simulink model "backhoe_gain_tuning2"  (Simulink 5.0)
settings: Solver=ode4  StartTime=0.0  StopTime=inf  FixedStep=0.001  RelTol=1e-3
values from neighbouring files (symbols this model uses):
  Butter_Order = 2    [startup.m]
  c1 = [-0.0009634 -0.4050766 2.3355377]    [startup.m]
  c2 = [ -0.00644514 2.23812750 22.79925627]    [startup.m]
  c3 = [-0.0057802 2.2376391 22.8266324]    [startup.m]
  c4 = [-0.0020828 1.5286223 20.3434998]    [startup.m]
undefined symbols (not defined in the file or in its folder): channels, ended, Single
libraries: dsparch4 x18, xpclib x6, simulink x1

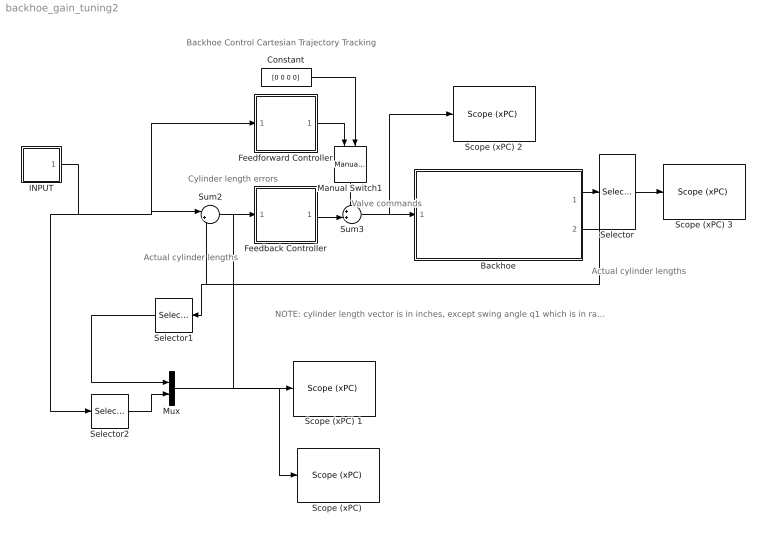
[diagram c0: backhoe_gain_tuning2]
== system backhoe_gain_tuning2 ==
  note: Backhoe Control Cartesian Trajectory Tracking
  note: NOTE: cylinder length vector is in inches, except swing angle q1 which is in radians: yc = [ q1[rad] yc,boom[in] yc,stick[in] yc,bucket[in] ]^T
  note: Cylinder length errors
  note: Actual cylinder lengths
  note: Actual cylinder lengths
  note: Valve commands
  Backhoe : Subsystem
  Constant : Constant  Value=[0 0 0 0]
  Feedback Controller : Subsystem
  Feedforward Controller : Subsystem
  INPUT : Subsystem
  Manual Switch1 : simulink/Signal Routing/Manual Switch  Orientation=down  sw=1  action=0
  Mux : Mux  Inputs=2
  "Scope (xPC) " : xpclib/Misc./Scope (xPC)   scopeno=1  scopetype=Target  viewmode=Graphical redraw  grid=on  ylimits=[0,40]  autostart=on  nosamples=2000  noprepostsamples=0  interleave=1  triggermode=FreeRun  triggersignal=1  triggerlevel=0.0  triggerslope=either  triggerscope=1  triggersample=0
  Scope (xPC) 1 : xpclib/Misc./Scope (xPC)   scopeno=2  scopetype=Target  viewmode=Graphical redraw  grid=on  ylimits=[-3,3]  autostart=on  nosamples=2000  noprepostsamples=0  interleave=1  triggermode=FreeRun  triggersignal=1  triggerlevel=0.0  triggerslope=either  triggerscope=1  triggersample=0
  Scope (xPC) 2 : xpclib/Misc./Scope (xPC)   scopeno=3  scopetype=Target  viewmode=Graphical redraw  grid=on  ylimits=[-1,1]  autostart=on  nosamples=2000  noprepostsamples=0  interleave=1  triggermode=FreeRun  triggersignal=1  triggerlevel=0.0  triggerslope=either  triggerscope=1  triggersample=0
  Scope (xPC) 3 : xpclib/Misc./Scope (xPC)   scopeno=4  scopetype=Target  viewmode=Graphical redraw  grid=on  ylimits=[0,1000]  autostart=on  nosamples=2000  noprepostsamples=0  interleave=1  triggermode=FreeRun  triggersignal=1  triggerlevel=0.0  triggerslope=either  triggerscope=1  triggersample=0
  Selector : Selector  Elements=[3 7]  InputPortWidth=10
  Selector1 : Selector  Orientation=left  Elements=[3]  InputPortWidth=4
  Selector2 : Selector  Elements=[3]  InputPortWidth=4
  Sum2 : Sum  Inputs=|+-
  Sum3 : Sum  Inputs=++|
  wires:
  Sum2/1 -> Feedback Controller/1(e), Scope (xPC) 1/1
  Backhoe/2(yc) -> Sum2/2, Selector1/1
  Feedback Controller/1(Us) -> Sum3/2
  Sum3/1 -> Backhoe/1(Us), Scope (xPC) 2/1
  Manual Switch1/1 -> Sum3/1
  Feedforward Controller/1(UsFF) -> Manual Switch1/1
  Constant/1 -> Manual Switch1/2
  Mux/1 -> "Scope (xPC) "/1
  Selector2/1 -> Mux/2
  Selector1/1 -> Mux/1
  INPUT/1(ycdes) -> Selector2/1, Sum2/1, Feedforward Controller/1(ycdes)
  Backhoe/1(Pres) -> Selector/1
  Selector/1 -> Scope (xPC) 3/1

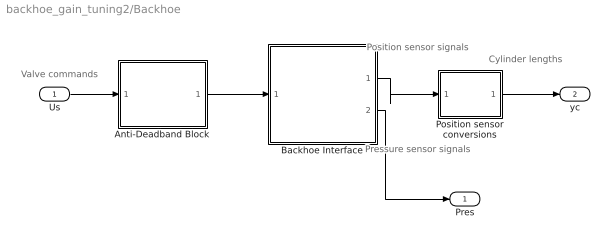
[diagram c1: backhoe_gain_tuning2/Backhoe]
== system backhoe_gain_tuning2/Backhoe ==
  note: Valve commands
  note: Position sensor signals
  note: Cylinder lengths
  note: Pressure sensor signals
  Us : Inport
  Anti-Deadband Block : Subsystem
  Backhoe Interface : Subsystem
  Position sensor conversions : Subsystem
  Pres : Outport
  yc : Outport  Port=2
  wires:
  Backhoe Interface/1(Vpos) -> Position sensor conversions/1(Vc)
  Position sensor conversions/1(yc) -> yc/1
  Us/1 -> Anti-Deadband Block/1(us)
  Backhoe Interface/2(Vpres) -> Pres/1
  Anti-Deadband Block/1(Us) -> Backhoe Interface/1(Us)

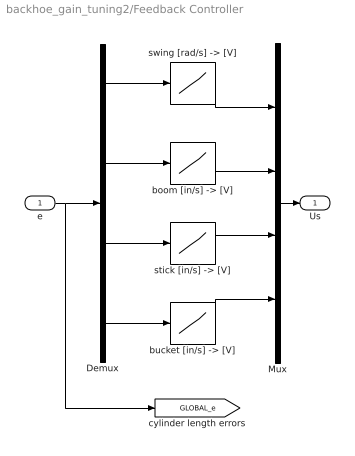
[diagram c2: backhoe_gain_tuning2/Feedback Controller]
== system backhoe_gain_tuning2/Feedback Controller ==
  e : Inport
  Demux : Demux
  Mux : Mux
  "boom [in/s] -> [V]" : Lookup  InputValues=[-1 0 1]  OutputValues=[-0.05 0 0.6]  ShowAdditionalParam=on
  "bucket [in/s] -> [V]" : Lookup  InputValues=[-1 0 1]  OutputValues=[-0.2 0 0.2]  ShowAdditionalParam=on
  "stick [in/s] -> [V]" : Lookup  InputValues=[-1 0 1]  OutputValues=[-0.2 0 0.2]  ShowAdditionalParam=on
  "swing [rad/s] -> [V]" : Lookup  InputValues=[-1 0 1]  OutputValues=[-0.2 0 0.2]  ShowAdditionalParam=on
  Us : Outport
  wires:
  e/1 -> [GLOBAL_e], Demux/1
  Demux/1 -> "swing [rad/s] -> [V]"/1
  "swing [rad/s] -> [V]"/1 -> Mux/1
  Demux/2 -> "boom [in/s] -> [V]"/1
  "boom [in/s] -> [V]"/1 -> Mux/2
  Demux/3 -> "stick [in/s] -> [V]"/1
  "stick [in/s] -> [V]"/1 -> Mux/3
  Demux/4 -> "bucket [in/s] -> [V]"/1
  "bucket [in/s] -> [V]"/1 -> Mux/4
  Mux/1 -> Us/1

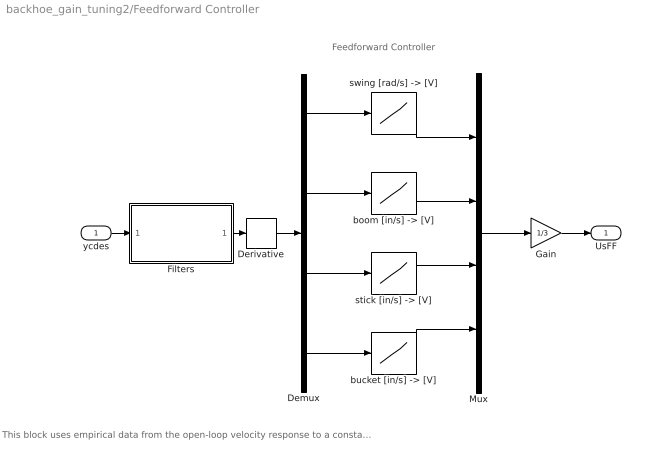
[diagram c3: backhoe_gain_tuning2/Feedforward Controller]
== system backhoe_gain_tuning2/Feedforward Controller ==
  note: This block uses empirical data from the open-loop velocity response to a constant voltage command to the valves. Relationships have been inverted to determine the required voltage to produce a desired velocity for each function.
  note: Feedforward Controller
  ycdes : Inport
  Demux : Demux
  Derivative : Derivative
  Filters : Subsystem
  Gain : Gain  Gain=1/3
  Mux : Mux
  "boom [in/s] -> [V]" : Lookup  InputValues=[-1.0 0 3.0]  OutputValues=[-0.25 0 0.25]  ShowAdditionalParam=on
  "bucket [in/s] -> [V]" : Lookup  InputValues=[-2.3 0 2.75]  OutputValues=[-0.25 0 0.25]  ShowAdditionalParam=on
  "stick [in/s] -> [V]" : Lookup  InputValues=[-1.6 0 1.75]  OutputValues=[-0.25 0 0.25]  ShowAdditionalParam=on
  "swing [rad/s] -> [V]" : Lookup  InputValues=[-0.6 0 0.7]  OutputValues=[-0.25 0 0.25]  ShowAdditionalParam=on
  UsFF : Outport
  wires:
  ycdes/1 -> Filters/1(unfiltered)
  Derivative/1 -> Demux/1
  Demux/1 -> "swing [rad/s] -> [V]"/1
  "swing [rad/s] -> [V]"/1 -> Mux/1
  Demux/2 -> "boom [in/s] -> [V]"/1
  "boom [in/s] -> [V]"/1 -> Mux/2
  Demux/3 -> "stick [in/s] -> [V]"/1
  "stick [in/s] -> [V]"/1 -> Mux/3
  Demux/4 -> "bucket [in/s] -> [V]"/1
  "bucket [in/s] -> [V]"/1 -> Mux/4
  Mux/1 -> Gain/1
  Filters/1(filtered) -> Derivative/1
  Gain/1 -> UsFF/1

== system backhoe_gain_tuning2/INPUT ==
  Boom : Sin  Amplitude=0  Bias=31  Frequency=2*pi*0.1  SampleTime=0
  Bucket : Sin  Amplitude=0  Bias=32  Frequency=2*pi*0.1  SampleTime=0
  Mux2 : Mux
  Stick : Sin  Amplitude=0  Bias=33  Frequency=2*pi*0.1  SampleTime=0
  Swing : Sin  Amplitude=0  Frequency=2*pi*0.1  SampleTime=0
  ycdes : Outport
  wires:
  Swing/1 -> Mux2/1
  Bucket/1 -> Mux2/4
  Stick/1 -> Mux2/3
  Boom/1 -> Mux2/2
  Mux2/1 -> ycdes/1

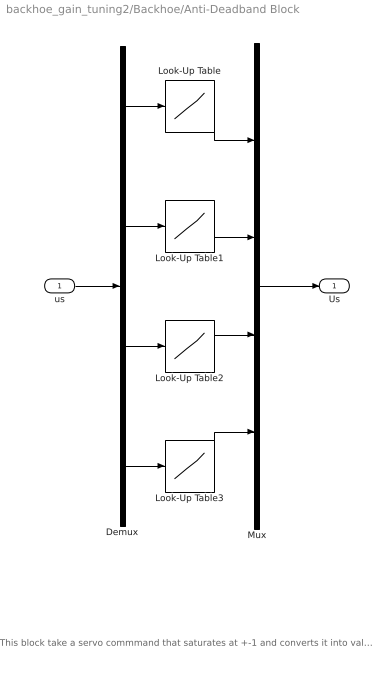
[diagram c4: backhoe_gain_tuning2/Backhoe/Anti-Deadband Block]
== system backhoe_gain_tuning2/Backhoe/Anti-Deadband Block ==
  note: This block take a servo commmand that saturates at +-1 and converts it into valve signals. "u" in the input signal which a 4-vector. Neutral is half the voltage supplied Vc to the valves which should 6V = 1/2 * 12V. Commands to the valve must be between 25% AND 75% of Vc where 50% is neutral or the "zero command" that tell the valve to stop flow to the valve. Neutral can either be set at 6V of measure from Channel 15.
  us : Inport
  Demux : Demux
  Look-Up Table{,1..3} (4 alike) : Lookup  InputValues=[-1 -0.02 0.02 1]  OutputValues=[3 5.45 6.55 9]  ShowAdditionalParam=on  LookUpMeth=Interpolation-Use End Values  OutDataTypeMode=double
  Mux : Mux
  Us : Outport
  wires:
  Look-Up Table/1 -> Mux/1
  Look-Up Table1/1 -> Mux/2
  Demux/1 -> Look-Up Table/1
  Demux/2 -> Look-Up Table1/1
  Demux/3 -> Look-Up Table2/1
  Look-Up Table2/1 -> Mux/3
  Demux/4 -> Look-Up Table3/1
  Look-Up Table3/1 -> Mux/4
  Mux/1 -> Us/1
  us/1 -> Demux/1

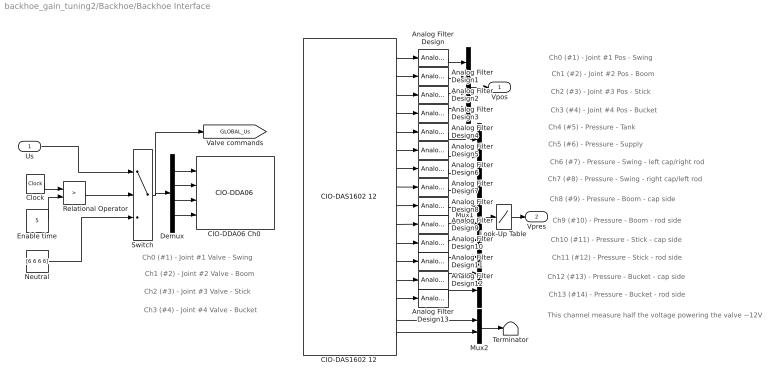
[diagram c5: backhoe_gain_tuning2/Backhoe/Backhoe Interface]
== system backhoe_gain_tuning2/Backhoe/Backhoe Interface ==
  note: Ch0 (#1) - Joint #1 Valve - Swing
  note: Ch1 (#2) - Joint #2 Valve - Boom
  note: Ch2 (#3) - Joint #3 Valve - Stick
  note: Ch3 (#4) - Joint #4 Valve - Bucket
  note: Ch0 (#1) - Joint #1 Pos - Swing
  note: Ch1 (#2) - Joint #2 Pos - Boom
  note: Ch2 (#3) - Joint #3 Pos - Stick
  note: Ch3 (#4) - Joint #4 Pos - Bucket
  note: Ch4 (#5) - Pressure - Tank
  note: Ch5 (#6) - Pressure - Supply
  note: Ch6 (#7) - Pressure - Swing - left cap/right rod
  note: Ch7 (#8) - Pressure - Swing - right cap/left rod
  note: Ch8 (#9) - Pressure - Boom - cap side
  note: Ch9 (#10) - Pressure - Boom - rod side
  note: Ch10 (#11) - Pressure - Stick - cap side
  note: Ch11 (#12) - Pressure - Stick - rod side
  note: Ch12 (#13) - Pressure - Bucket - cap side
  note: Ch13 (#14) - Pressure - Bucket - rod side
  note: This channel measure half the voltage powering the valve ~12V
  Us : Inport
  Analog Filter Design{,1..13} (14 alike) : dsparch4/Analog Filter Design  method=Butterworth  filttype=Lowpass  N=Butter_Order  Wlo=Butter_Rad  Whi=80  Rp=2  Rs=40
  "CIO-DAS1602 12 " : xpclib/A//D/Computer Boards/CIO-DAS1602 12   channel=16  range=0-10V  mux=Single-ended (16 channels)  sampletime=0.001  baseaddress=0x340
  "CIO-DDA06 Ch0 " : xpclib/D//A/Computer Boards/CIO-DDA06   channel=[1 2 3 4]  range=[10 10 10 10]  reset=[1 1 1 1]  initValue=[6 6 6 6]  sampletime=0.001  baseaddress=0x300
  Clock : Clock
  Demux : Demux
  Enable time : Constant  Value=5
  Look-Up Table : Lookup  InputValues=[2 10]  OutputValues=[0 3000]
  Mux : Mux
  Mux1 : Mux  Inputs=10
  Mux2 : Mux  Inputs=2
  Neutral : Constant  Value=[6 6 6 6]  ShowAdditionalParam=on
  Relational Operator : RelationalOperator  Operator=>  ShowAdditionalParam=on
  Switch : Switch  Threshold=0.5  ShowAdditionalParam=on
  Terminator : Terminator
  Vpos : Outport
  Vpres : Outport  Port=2
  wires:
  Demux/1 -> "CIO-DDA06 Ch0 "/1
  Demux/2 -> "CIO-DDA06 Ch0 "/2
  Demux/3 -> "CIO-DDA06 Ch0 "/3
  Demux/4 -> "CIO-DDA06 Ch0 "/4
  Mux/1 -> Vpos/1
  "CIO-DAS1602 12 "/1 -> Analog Filter Design/1
  Analog Filter Design/1 -> Mux/1
  "CIO-DAS1602 12 "/2 -> Analog Filter Design1/1
  "CIO-DAS1602 12 "/3 -> Analog Filter Design2/1
  "CIO-DAS1602 12 "/4 -> Analog Filter Design3/1
  Analog Filter Design1/1 -> Mux/2
  Analog Filter Design2/1 -> Mux/3
  Analog Filter Design3/1 -> Mux/4
  "CIO-DAS1602 12 "/5 -> Analog Filter Design4/1
  "CIO-DAS1602 12 "/6 -> Analog Filter Design5/1
  "CIO-DAS1602 12 "/7 -> Analog Filter Design6/1
  "CIO-DAS1602 12 "/8 -> Analog Filter Design7/1
  "CIO-DAS1602 12 "/9 -> Analog Filter Design8/1
  "CIO-DAS1602 12 "/10 -> Analog Filter Design9/1
  "CIO-DAS1602 12 "/11 -> Analog Filter Design10/1
  "CIO-DAS1602 12 "/12 -> Analog Filter Design11/1
  "CIO-DAS1602 12 "/13 -> Analog Filter Design12/1
  "CIO-DAS1602 12 "/14 -> Analog Filter Design13/1
  "CIO-DAS1602 12 "/15 -> Mux2/1
  Analog Filter Design4/1 -> Mux1/1
  Analog Filter Design5/1 -> Mux1/2
  Analog Filter Design6/1 -> Mux1/3
  Analog Filter Design7/1 -> Mux1/4
  Analog Filter Design8/1 -> Mux1/5
  Analog Filter Design9/1 -> Mux1/6
  Analog Filter Design10/1 -> Mux1/7
  Analog Filter Design11/1 -> Mux1/8
  Analog Filter Design12/1 -> Mux1/9
  Analog Filter Design13/1 -> Mux1/10
  Mux2/1 -> Terminator/1
  "CIO-DAS1602 12 "/16 -> Mux2/2
  Switch/1 -> Demux/1, [GLOBAL_Us]
  Clock/1 -> Relational Operator/1
  Enable time/1 -> Relational Operator/2
  Relational Operator/1 -> Switch/2
  Neutral/1 -> Switch/3
  Us/1 -> Switch/1
  Look-Up Table/1 -> Vpres/1
  Mux1/1 -> Look-Up Table/1

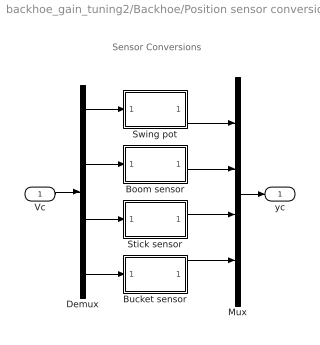
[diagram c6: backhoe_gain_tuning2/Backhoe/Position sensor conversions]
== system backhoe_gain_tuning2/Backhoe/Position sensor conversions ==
  note: Sensor Conversions
  Vc : Inport
  Boom sensor : Subsystem
  Bucket sensor : Subsystem
  Demux : Demux
  Mux : Mux
  Stick sensor : Subsystem
  Swing pot : Subsystem
  yc : Outport
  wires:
  Vc/1 -> Demux/1
  Demux/1 -> Swing pot/1(Vc1)
  Demux/2 -> Boom sensor/1(Vc2)
  Swing pot/1(q1) -> Mux/1
  Boom sensor/1(yc3) -> Mux/2
  Demux/3 -> Stick sensor/1(Vc3)
  Stick sensor/1(yc4) -> Mux/3
  Mux/1 -> yc/1
  Demux/4 -> Bucket sensor/1(Vc4)
  Bucket sensor/1(yc5) -> Mux/4

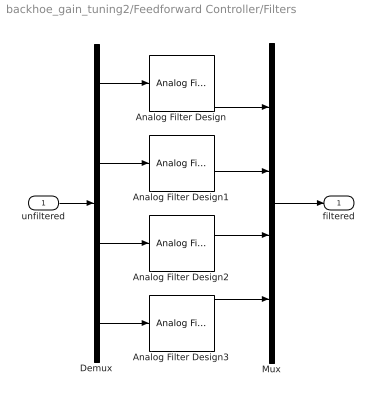
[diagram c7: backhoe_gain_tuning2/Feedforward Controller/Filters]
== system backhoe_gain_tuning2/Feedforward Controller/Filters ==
  unfiltered : Inport
  Analog Filter Design{,1..3} (4 alike) : dsparch4/Analog Filter Design  method=Butterworth  filttype=Lowpass  N=2  Wlo=2*pi*5  Whi=80  Rp=2  Rs=40
  Demux : Demux
  Mux : Mux
  filtered : Outport
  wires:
  unfiltered/1 -> Demux/1
  Demux/1 -> Analog Filter Design/1
  Analog Filter Design/1 -> Mux/1
  Demux/2 -> Analog Filter Design1/1
  Analog Filter Design1/1 -> Mux/2
  Demux/3 -> Analog Filter Design2/1
  Analog Filter Design2/1 -> Mux/3
  Demux/4 -> Analog Filter Design3/1
  Analog Filter Design3/1 -> Mux/4
  Mux/1 -> filtered/1

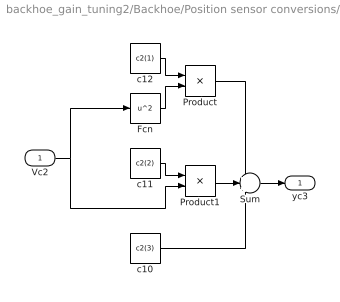
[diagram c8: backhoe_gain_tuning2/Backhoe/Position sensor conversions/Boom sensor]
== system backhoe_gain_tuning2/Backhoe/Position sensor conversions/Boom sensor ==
  Vc2 : Inport
  Fcn : Fcn  Expr=u^2
  Product : Product
  Product1 : Product
  Sum : Sum  Inputs=+++
  c10 : Constant  Value=c2(3)
  c11 : Constant  Value=c2(2)
  c12 : Constant  Value=c2(1)
  yc3 : Outport
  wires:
  Vc2/1 -> Fcn/1, Product1/2
  Product1/1 -> Sum/2
  c10/1 -> Sum/3
  c12/1 -> Product/1
  Fcn/1 -> Product/2
  Product/1 -> Sum/1
  c11/1 -> Product1/1
  Sum/1 -> yc3/1

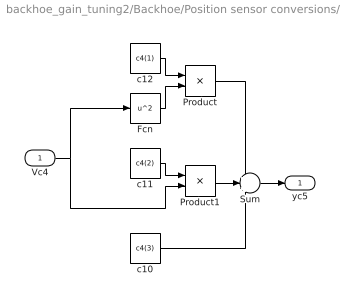
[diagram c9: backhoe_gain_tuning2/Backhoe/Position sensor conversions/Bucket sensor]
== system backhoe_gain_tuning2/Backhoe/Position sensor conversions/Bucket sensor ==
  Vc4 : Inport
  Fcn : Fcn  Expr=u^2
  Product : Product
  Product1 : Product
  Sum : Sum  Inputs=+++
  c10 : Constant  Value=c4(3)
  c11 : Constant  Value=c4(2)
  c12 : Constant  Value=c4(1)
  yc5 : Outport
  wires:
  Vc4/1 -> Fcn/1, Product1/2
  Product1/1 -> Sum/2
  c10/1 -> Sum/3
  c12/1 -> Product/1
  Fcn/1 -> Product/2
  Product/1 -> Sum/1
  c11/1 -> Product1/1
  Sum/1 -> yc5/1

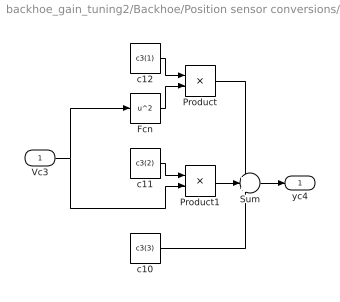
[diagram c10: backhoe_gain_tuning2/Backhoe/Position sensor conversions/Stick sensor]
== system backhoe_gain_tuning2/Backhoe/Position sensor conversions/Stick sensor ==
  Vc3 : Inport
  Fcn : Fcn  Expr=u^2
  Product : Product
  Product1 : Product
  Sum : Sum  Inputs=+++
  c10 : Constant  Value=c3(3)
  c11 : Constant  Value=c3(2)
  c12 : Constant  Value=c3(1)
  yc4 : Outport
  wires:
  Vc3/1 -> Fcn/1, Product1/2
  Product1/1 -> Sum/2
  c10/1 -> Sum/3
  c12/1 -> Product/1
  Fcn/1 -> Product/2
  Product/1 -> Sum/1
  c11/1 -> Product1/1
  Sum/1 -> yc4/1

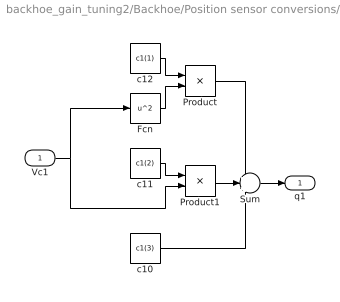
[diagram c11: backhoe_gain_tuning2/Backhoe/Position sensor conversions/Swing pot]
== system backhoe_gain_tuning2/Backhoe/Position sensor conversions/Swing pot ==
  Vc1 : Inport
  Fcn : Fcn  Expr=u^2
  Product : Product
  Product1 : Product
  Sum : Sum  Inputs=+++
  c10 : Constant  Value=c1(3)
  c11 : Constant  Value=c1(2)
  c12 : Constant  Value=c1(1)
  q1 : Outport
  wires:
  Vc1/1 -> Fcn/1, Product1/2
  Product1/1 -> Sum/2
  c10/1 -> Sum/3
  c12/1 -> Product/1
  Fcn/1 -> Product/2
  Product/1 -> Sum/1
  c11/1 -> Product1/1
  Sum/1 -> q1/1
